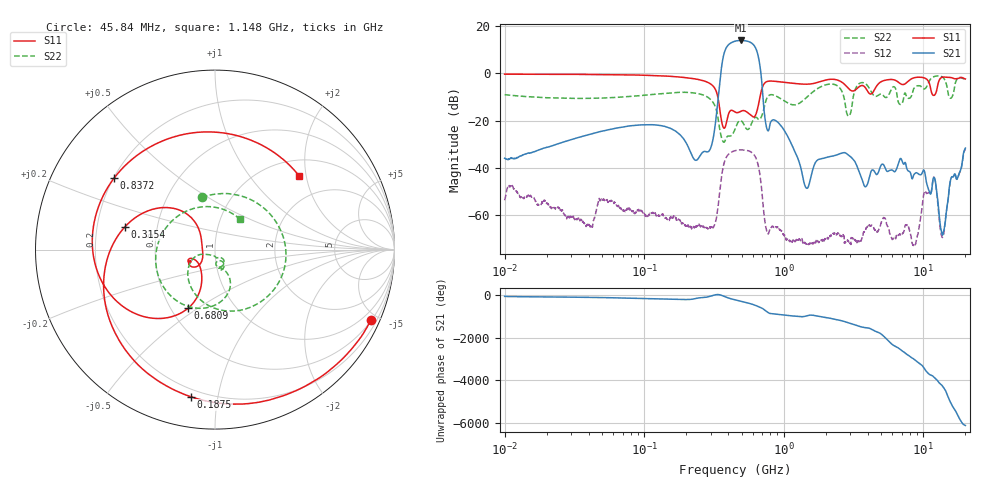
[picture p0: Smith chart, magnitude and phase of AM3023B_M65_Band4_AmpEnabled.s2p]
!Agilent Technologies,E8364B,MY43040894,A.07.50.67
!Agilent E8364B: A.07.50.67
!Date: Tuesday, October 27, 2020 10:53:07
!Correction: S11(Full 2 Port(1,2))
!S21(Full 2 Port(1,2))
!S12(Full 2 Port(1,2))
!S22(Full 2 Port(1,2))
!S2P File: Measurements: S11, S21, S12, S22:Log Frequency Sweep
# Hz S  dB  R 50
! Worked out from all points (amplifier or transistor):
!   3201 points, 10 MHz to 20 GHz, reference 50 ohm
!   highest |S21| = 14.0 dB at 493 MHz (marker M1)
!   |S21| within 3 dB of that: 387.9 MHz to 625.8 MHz (237.9 MHz wide, 46.9 % of centre)
!   unconditionally stable (mu >= 1): start of sweep to end of sweep
!   at 35.47 MHz: K = 1068.92, MAG = -15.6 dB, |S12| = -62.1 dB
!   at 447.2 MHz: K = 4.40, MAG = 13.8 dB, |S12| = -32.7 dB
!   at 20 GHz: K = 140.25, MAG = -24.3 dB, |S12| = -32.0 dB
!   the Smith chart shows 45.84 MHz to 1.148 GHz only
!   S11 on the Smith chart (normalised r, x): 45.84 MHz: 0.53, -4.60; 187.5 MHz: 0.16, -0.84; 315.4 MHz: 0.32, +0.11; 680.9 MHz: 0.61, -0.46; 837.2 MHz: 0.20, +0.31; 1.148 GHz: 1.35, +1.82
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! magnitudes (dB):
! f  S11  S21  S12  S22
! 10 MHz  -0.3  -35.9  -53.6  -9.0
! 35.55 MHz  -0.4  -26.7  -62.1  -10.5
! 45.84 MHz  -0.4  -25.0  -57.0  -10.4
! 126.1 MHz  -0.9  -21.9  -60.3  -8.7
! 187.5 MHz  -1.6  -26.9  -63.2  -7.9
! 235.5 MHz  -2.4  -36.7  -64.7  -8.4
! 315.4 MHz  -5.7  -25.9  -64.8  -12.8
! 370.7 MHz  -23.0  7.7  -38.7  -29.1
! 447.2 MHz  -16.3  13.7  -32.7  -23.5
! 493 MHz  -16.0  14.0  -32.3  -20.0
! 680.9 MHz  -8.9  1.5  -44.7  -19.0
! 752.4 MHz  -3.5  -22.8  -66.2  -10.8
! 837.2 MHz  -3.2  -19.6  -64.9  -9.1
! 1.148 GHz  -4.1  -30.5  -71.1  -13.2
! 1.439 GHz  -4.5  -48.3  -72.0  -10.4
! 1.59 GHz  -4.3  -42.0  -71.9  -8.1
! 5.639 GHz  -2.6  -41.2  -65.6  -9.1
! 8.647 GHz  -1.8  -42.5  -72.8  -5.9
! 11.92 GHz  -9.3  -44.0  -43.9  -1.3
! 13.74 GHz  -1.5  -68.3  -69.3  -1.6
! 15.81 GHz  -1.7  -44.2  -44.2  -10.4
! 20 GHz  -2.3  -31.6  -32.0  -2.6
